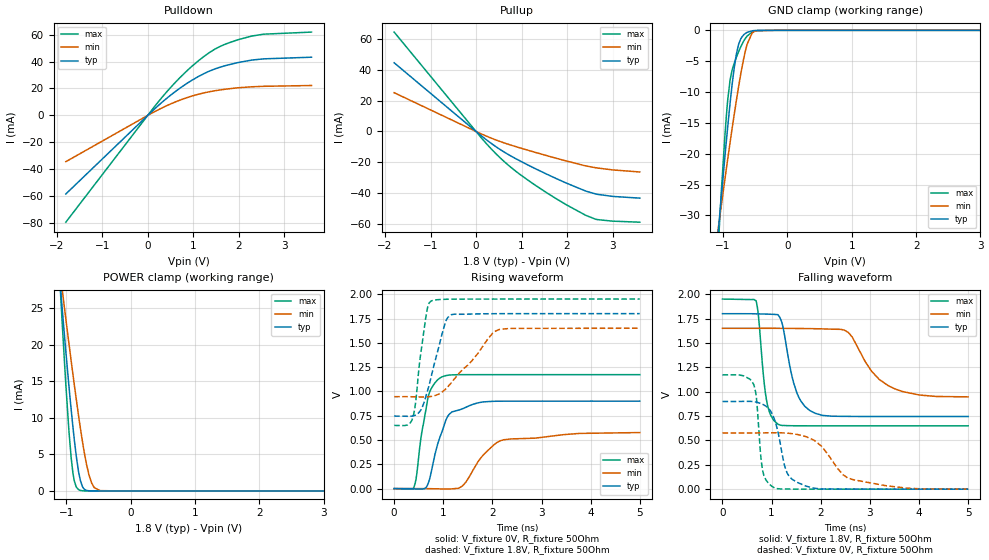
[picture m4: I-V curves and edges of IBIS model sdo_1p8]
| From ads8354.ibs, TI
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|   sdo_1p8 Model
[Model]   sdo_1p8
Model_type   3-state
Polarity   Non-Inverting
Vmeas = 0.9
Vref = 0
Cref = 10pF
Rref = 150
|   typ   min   max
|   (nom PVT)   (fast PVT)   (slow PVT)
C_comp   1.236e-12   9.672e-13   1.523e-12
| Where nom  PVT is Nominal Process, 1.8V, 27C
|   Fast PVT is Strong Process,  1.95V, -40C
|   Slow PVT is Weak Process,   1.65V, 125C
[Voltage Range]   1.8   1.65   1.95
|Junction Temperature
[Temperature Range]   27   125   -40
[Pullup Reference]   1.8   1.65   1.95
[Pulldown Reference]   0   0   0
[Power Clamp Reference]   1.8   1.65   1.95
[GND Clamp Reference]   0   0   0
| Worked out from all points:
|   slope of the pulldown table from 0 to 0.27 V, typ, clamps not added: 32 ohm
|   slope of the pullup table from 0 to 0.27 V, typ, clamps not added: 42.7 ohm
|   GND clamp passes 1 mA (typ) near -0.70 V on its own axis
|   POWER clamp passes 1 mA (typ) near -0.77 V on its own axis
|   falling waveform, V_fixture 1.8V, R_fixture 50Ohm: 20-80 % time 282ps typ, 605ps min, 149ps max; typ from 1.8 V to 0.745 V
|   rising waveform, V_fixture 0V, R_fixture 50Ohm: 20-80 % time 308ps typ, 537ps min, 210ps max; typ from 0 V to 0.9 V
|   rising waveform, V_fixture 1.8V, R_fixture 50Ohm: 20-80 % time 323ps typ, 706ps min, 182ps max; typ from 0.745 V to 1.8 V
|   falling waveform, V_fixture 0V, R_fixture 50Ohm: 20-80 % time 249ps typ, 581ps min, 114ps max; typ from 0.9 V to 0 V
[Pulldown]
|   Voltage   I(typ)   I(min)   I(max)
-1.8V     -58.29mA   -34.32mA   -79.21mA
302.1mV   9.381mA    5.377mA    12.89mA
569.3mV   16.74mA    9.463mA    23.14mA
846.1mV   23.4mA     13mA       32.58mA
1.242V    31.1mA     16.77mA    43.9mA
1.472V    34.43mA    18.28mA    49.09mA
1.657V    36.45mA    19.22mA    52.17mA
1.979V    39.18mA    20.48mA    56.1mA
2.285V    41.05mA    21.24mA    58.88mA
2.548V    41.97mA    21.6mA     60.28mA
3.6V      43.19mA    22.19mA    61.83mA
[GND Clamp]
|   Voltage   I(typ)   I(min)   I(max)
-1.8V     -126.5mA   -91.53mA   -183mA
-1.085V   -33.96mA   -32.94mA   -36.86mA
-1.03V    -27.25mA   -28.6mA    -26.67mA
-948.6mV  -17.92mA   -22.44mA   -13.86mA
-893.2mV  -12.05mA   -18.36mA   -8.262mA
-829.8mV  -6.32mA    -13.86mA   -5.433mA
-763.2mV  -2.451mA   -9.428mA   -3.589mA
-709.4mV  -1.111mA   -6.188mA   -2.329mA
-626.9mV  -334.7uA   -2.276mA   -937.8uA
-551mV    -87.72uA   -489.9uA   -295.6uA
-463.5mV  -12.09uA   -49.05uA   -43.83uA
3.6V      0A         0A         0A
[Pullup]
|   Voltage   I(typ)   I(min)   I(max)
-1.8V     44.36mA    25.04mA    64.18mA
200.7mV   -4.776mA   -2.66mA    -6.968mA
511.2mV   -11.3mA    -6.286mA   -16.49mA
843.3mV   -17.09mA   -9.501mA   -24.98mA
1.211V    -22.69mA   -12.72mA   -32.88mA
1.624V    -28.54mA   -16.18mA   -40.9mA
1.982V    -33.29mA   -19.06mA   -47.29mA
2.41V     -38.49mA   -22.24mA   -54.13mA
2.665V    -40.57mA   -23.59mA   -56.92mA
3.033V    -42.01mA   -24.9mA    -57.96mA
3.6V      -43.06mA   -26.16mA   -58.59mA
[POWER Clamp]
|   Voltage   I(typ)   I(min)   I(max)
-1.8V     109mA      84.85mA    147.1mA
-1.105V   29.27mA    30.48mA    29.33mA
-1.063V   24.7mA     27.4mA     22.64mA
-1.028V   21.02mA    24.89mA    17.33mA
-963.5mV  14.63mA    20.38mA    8.577mA
-924.4mV  11.01mA    17.71mA    4.433mA
-874.8mV  6.827mA    14.39mA    1.296mA
-805.1mV  2.352mA    9.942mA    145.9uA
-734.1mV  358.2uA    5.879mA    12.84uA
-648mV    16.6uA     2.149mA    728.9nA
-478.3mV  40.5nA     41.84uA    0A
3.6V      0A         0A         0A
[Ramp]
R_load = 50
|   typ   min   max
dV/dt_r   0.539745/3.07107e-10   0.345837/5.35968e-10   0.703331/2.09672e-10
dV/dt_f   0.632829/2.81125e-10   0.421998/5.90776e-10   0.780205/1.49062e-10
[Falling Waveform]
V_fixture = 1.8V
V_fixture_min = 1.65V
V_fixture_max = 1.95V
R_fixture = 50Ohm
|   Time   V(typ)   V(min)   V(max)
0s        1.8V       1.65V      1.95V
683ps     1.798V     1.65V      1.933V
895ps     1.796V     1.65V      917mV
1.126ns   1.79V      1.65V      667.4mV
1.512ns   992mV      1.648V     650.3mV
1.779ns   806.3mV    1.647V     650mV
2.562ns   746.4mV    1.607V     649.7mV
3.036ns   745.5mV    1.209V     649.7mV
3.517ns   745.4mV    1.027V     649.7mV
5ns       745.3mV    946.7mV    649.7mV
[Rising Waveform]
V_fixture = 0V
V_fixture_min = 0V
V_fixture_max = 0V
R_fixture = 50Ohm
|   Time   V(typ)   V(min)   V(max)
0s        1.017nV    3.484nV    831.6pV
403.5ps   -2.731mV   286.1uV    13.76mV
558ps     -4.731mV   103.8uV    563.2mV
695ps     56.18mV    -715.8uV   948.9mV
971ps     580.6mV    -3.395mV   1.149V
1.177ns   789.1mV    -2.999mV   1.17V
1.405ns   823.9mV    33.62mV    1.172V
1.829ns   892.2mV    353.7mV    1.172V
2.231ns   899.2mV    502.2mV    1.172V
5ns       899.6mV    576.4mV    1.172V
[Rising Waveform]
V_fixture = 1.8V
V_fixture_min = 1.65V
V_fixture_max = 1.95V
R_fixture = 50Ohm
|   Time   V(typ)   V(min)   V(max)
0s        745.3mV    945.4mV    649.7mV
277.5ps   743.6mV    945.6mV    654.8mV
385ps     747.4mV    944.6mV    737.5mV
538.5ps   805.2mV    942.4mV    1.38V
640.5ps   939.5mV    942.6mV    1.749V
753.5ps   1.151V     948mV      1.931V
1.044ns   1.711V     1.022V     1.948V
1.167ns   1.79V      1.091V     1.949V
2.146ns   1.8V       1.638V     1.95V
5ns       1.8V       1.65V      1.95V
[Falling Waveform]
V_fixture = 0V
V_fixture_min = 0V
V_fixture_max = 0V
R_fixture = 50Ohm
|   Time   V(typ)   V(min)   V(max)
0s        899.6mV    576.6mV    1.172V
636ps     897.4mV    576.7mV    1.073V
690ps     892.4mV    576.8mV    938mV
770.5ps   880.6mV    577.1mV    387.1mV
822.5ps   869.4mV    577.3mV    179.6mV
1.055ns   720.5mV    578.4mV    14.29mV
1.32ns    163.1mV    574.5mV    1.275mV
1.684ns   34.67mV    540.8mV    335uV
2.545ns   582uV      115.9mV    79.96uV
5ns       13.68uV    421.9uV    1.538uV
